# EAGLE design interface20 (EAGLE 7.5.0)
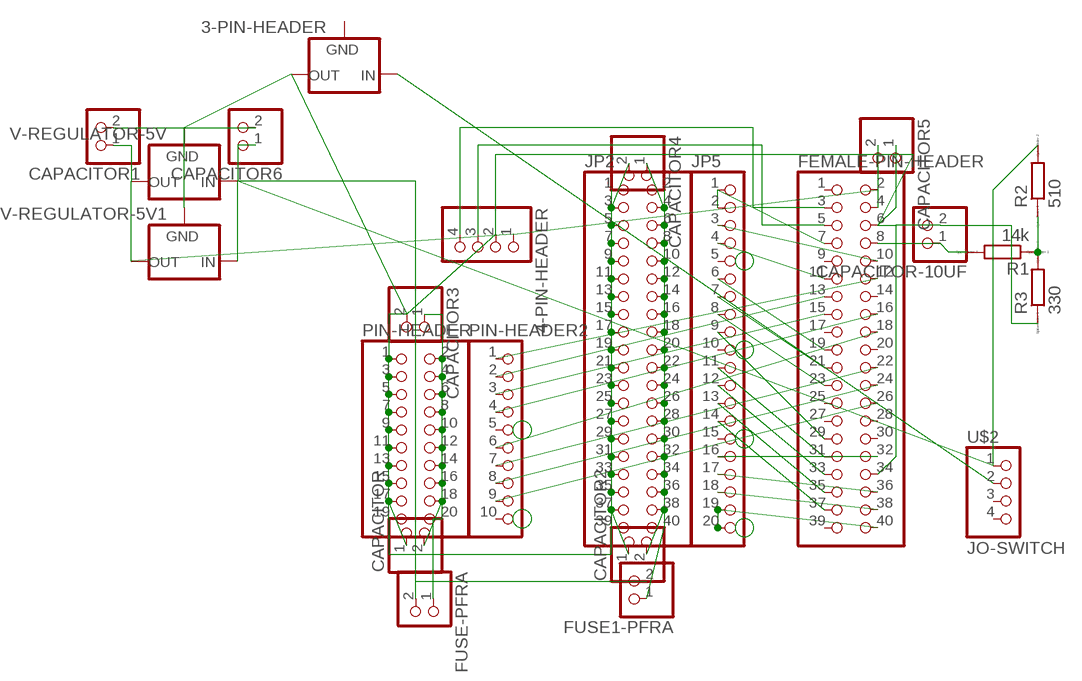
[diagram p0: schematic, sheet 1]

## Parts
3-PIN-HEADER  78MXXS  [78MXXS]
4-PIN-HEADER  PINHD-1X4  [1X04]
CAPACITOR  PINHD-1X2  [1X02]
CAPACITOR1  PINHD-1X2  [1X02]
CAPACITOR2  PINHD-1X2  [1X02]
CAPACITOR3  PINHD-1X2  [1X02]
CAPACITOR4  PINHD-1X2  [1X02]
CAPACITOR5  PINHD-1X2  [1X02]
CAPACITOR6  PINHD-1X2  [1X02]
CAPACITOR-10UF  PINHD-1X2  [1X02]
FEMALE-PIN-HEADER  PINHD-2X20  [2X20]
FUSE1-PFRA  PINHD-1X2  [1X02]
FUSE-PFRA  PINHD-1X2  [1X02]
JP2  PINHD-2X20  [2X20]
JP5  PINHD-1X20  [1X20]
PIN-HEADER  PINHD-2X10  [2X10]
PIN-HEADER2  PINHD-1X10  [1X10]
R1  14k  R0204/7  [0204/7]
R2  510  R0204/7  [0204/7]
R3  330  R0204/7  [0204/7]
U$2  JO-SWITCH  [JO-SWICH]
V-REGULATOR-5V  78MXXS  [78MXXS]
V-REGULATOR-5V1  78MXXS  [78MXXS]

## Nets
N$1 [dicker]: 3-PIN-HEADER.IN U$2.2
N$2: CAPACITOR-10UF.1 FEMALE-PIN-HEADER.8 R1.2
N$4: R1.1 R2.1 R3.2
N$7: 4-PIN-HEADER.4 FEMALE-PIN-HEADER.3
N$8: 4-PIN-HEADER.3 FEMALE-PIN-HEADER.5
N$9: FEMALE-PIN-HEADER.7 JP5.1 JP5.2
N$10: FEMALE-PIN-HEADER.10 JP5.3
N$11: FEMALE-PIN-HEADER.13 PIN-HEADER2.2
N$12: FEMALE-PIN-HEADER.11 JP5.4
N$13: FEMALE-PIN-HEADER.19 JP5.6
N$14: FEMALE-PIN-HEADER.21 JP5.7
N$15: FEMALE-PIN-HEADER.23 JP5.8
N$16: FEMALE-PIN-HEADER.29 JP5.9
N$17: FEMALE-PIN-HEADER.31 JP5.11
N$18: FEMALE-PIN-HEADER.33 JP5.12
N$19: FEMALE-PIN-HEADER.35 JP5.13
N$20: FEMALE-PIN-HEADER.37 JP5.14
N$21: FEMALE-PIN-HEADER.40 JP5.19 JP5.20
N$22: FEMALE-PIN-HEADER.38 JP5.18
N$23: FEMALE-PIN-HEADER.36 JP5.17
N$24: FEMALE-PIN-HEADER.32 JP5.16
N$25: FEMALE-PIN-HEADER.26 PIN-HEADER2.9
N$26: FEMALE-PIN-HEADER.24 PIN-HEADER2.8
N$27: FEMALE-PIN-HEADER.22 PIN-HEADER2.7
N$28: FEMALE-PIN-HEADER.18 PIN-HEADER2.6
N$29: FEMALE-PIN-HEADER.16 PIN-HEADER2.4
N$30: FEMALE-PIN-HEADER.12 PIN-HEADER2.1
N$31: FEMALE-PIN-HEADER.15 PIN-HEADER2.3
N$32 [mittel]: 4-PIN-HEADER.1 CAPACITOR1.1 CAPACITOR5.2 FEMALE-PIN-HEADER.2 FEMALE-PIN-HEADER.4 V-REGULATOR-5V1.OUT V-REGULATOR-5V.OUT
N$33 [dicker]: 3-PIN-HEADER.OUT 4-PIN-HEADER.2 CAPACITOR1.2 CAPACITOR2.1 CAPACITOR3.2 CAPACITOR4.2 CAPACITOR5.1 CAPACITOR6.2 CAPACITOR-10UF.2 CAPACITOR.1 FEMALE-PIN-HEADER.6 FEMALE-PIN-HEADER.34 JP2.1 JP2.3 JP2.5 JP2.7 JP2.9 JP2.11 JP2.13 JP2.15 JP2.17 JP2.19 JP2.21 JP2.23 JP2.25 JP2.27 JP2.29 JP2.31 JP2.33 JP2.35 JP2.37 JP2.39 PIN-HEADER.1 PIN-HEADER.3 PIN-HEADER.5 PIN-HEADER.7 PIN-HEADER.9 PIN-HEADER.11 PIN-HEADER.13 PIN-HEADER.15 PIN-HEADER.17 PIN-HEADER.19 R3.1 V-REGULATOR-5V1.GND V-REGULATOR-5V.GND
N$35 [dicker]: CAPACITOR2.2 CAPACITOR4.1 FUSE1-PFRA.1 JP2.2 JP2.4 JP2.6 JP2.8 JP2.10 JP2.12 JP2.14 JP2.16 JP2.18 JP2.20 JP2.22 JP2.24 JP2.26 JP2.28 JP2.30 JP2.32 JP2.34 JP2.36 JP2.38 JP2.40
N$36 [dicker]: CAPACITOR6.1 FUSE1-PFRA.2 FUSE-PFRA.2 R2.2 U$2.1 V-REGULATOR-5V1.IN V-REGULATOR-5V.IN
N$37 [dicker]: CAPACITOR3.1 CAPACITOR.2 FUSE-PFRA.1 PIN-HEADER.2 PIN-HEADER.4 PIN-HEADER.6 PIN-HEADER.8 PIN-HEADER.10 PIN-HEADER.12 PIN-HEADER.14 PIN-HEADER.16 PIN-HEADER.18 PIN-HEADER.20
Unconnected: 3-PIN-HEADER.GND FEMALE-PIN-HEADER.1 FEMALE-PIN-HEADER.9 FEMALE-PIN-HEADER.14 FEMALE-PIN-HEADER.17 FEMALE-PIN-HEADER.20 FEMALE-PIN-HEADER.25 FEMALE-PIN-HEADER.27 FEMALE-PIN-HEADER.28 FEMALE-PIN-HEADER.30 FEMALE-PIN-HEADER.39 JP5.5 JP5.10 JP5.15 PIN-HEADER2.5 PIN-HEADER2.10 U$2.3 U$2.4

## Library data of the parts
3-PIN-HEADER V-REGULATOR-5V V-REGULATOR-5V1 = v-reg:78MXXS: VOLTAGE REGULATOR
4-PIN-HEADER = pinhead:PINHD-1X4: PIN HEADER
CAPACITOR CAPACITOR1-CAPACITOR6 CAPACITOR-10UF FUSE1-PFRA FUSE-PFRA = pinhead:PINHD-1X2: PIN HEADER
FEMALE-PIN-HEADER JP2 = pinhead:PINHD-2X20: PIN HEADER
JP5 = pinhead:PINHD-1X20: PIN HEADER
PIN-HEADER = pinhead:PINHD-2X10: PIN HEADER
PIN-HEADER2 = pinhead:PINHD-1X10: PIN HEADER
R1-R3 = eagle-ltspice:R: RESISTOR, European symbol; SPICEMODEL: NONE; SPICEPREFIX: R
U$2 = pinhead:JO-SWITCH

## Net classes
1 dicker: width 1.27 mm, drill 1.016 mm, clearance 0.127 mm
2 mittel: width 0.508 mm, drill 0.508 mm

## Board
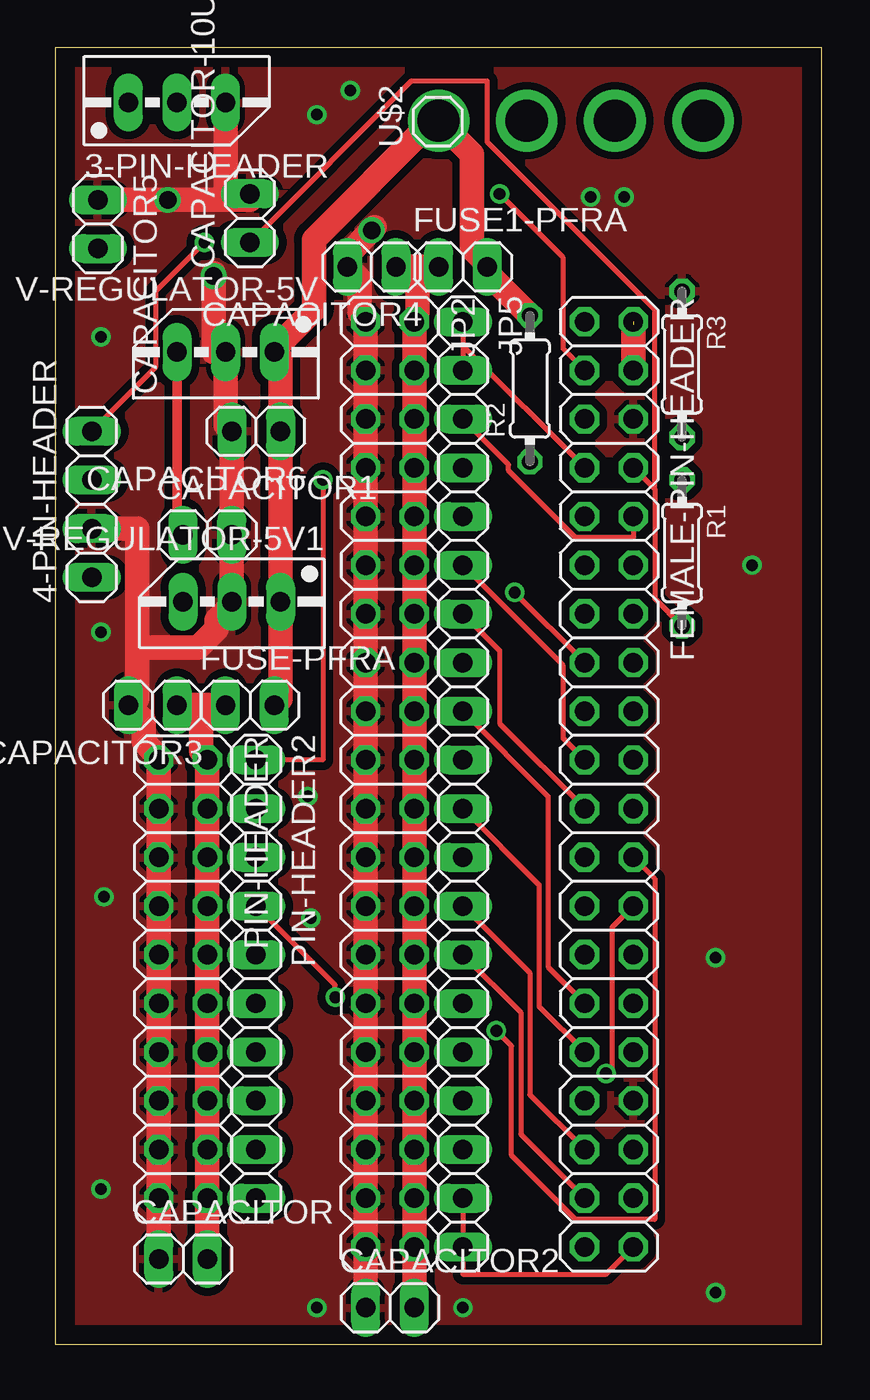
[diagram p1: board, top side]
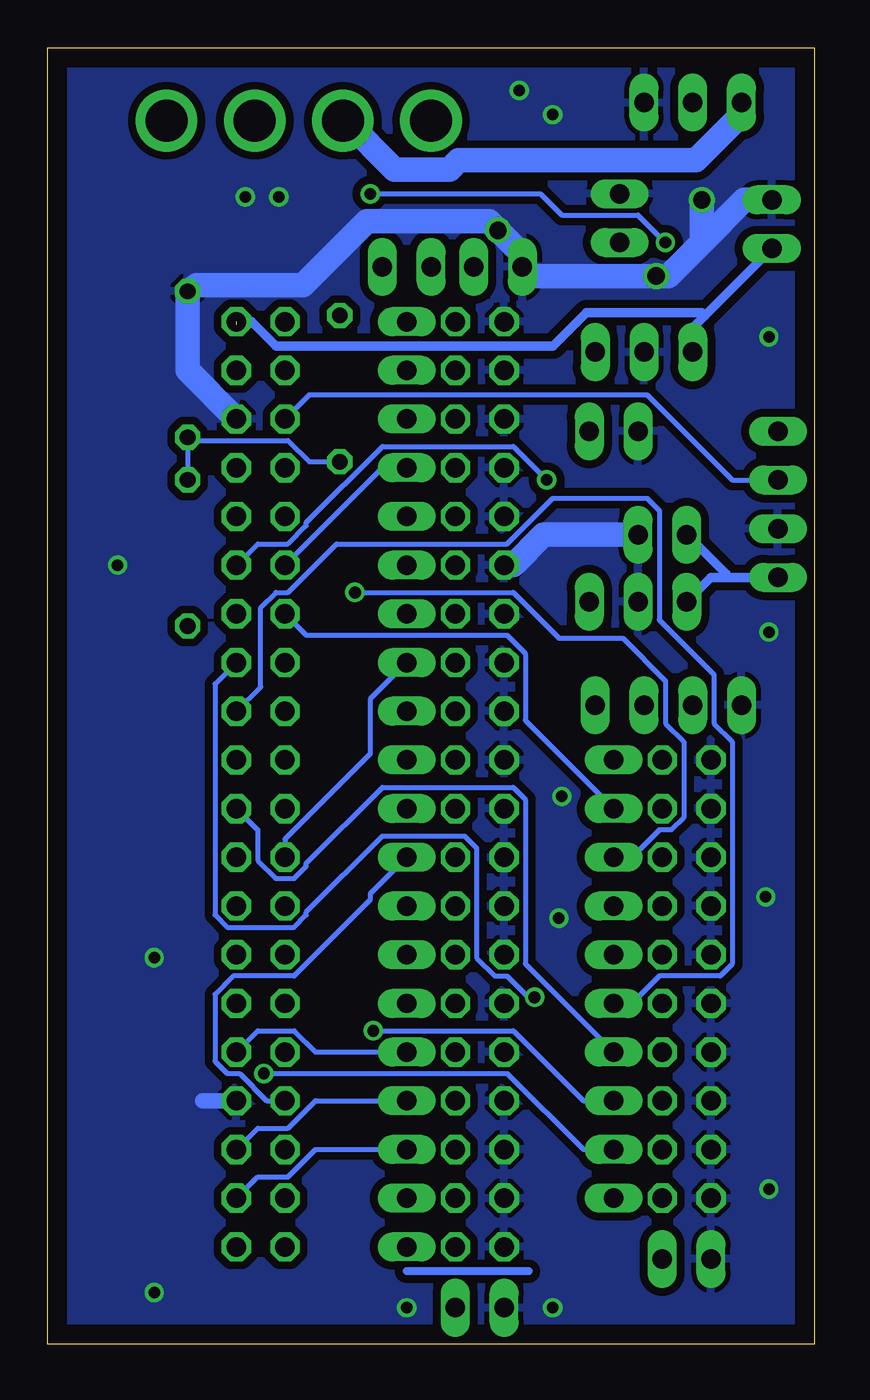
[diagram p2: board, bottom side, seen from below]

Size 39.99 x 67.62 mm. Coordinates in mm from the lower left corner, seen from the top.
Outline: 0,0 39.99,0 39.99,67.62 0,67.62 0,0
Copper layers (1*16): Top 0.035mm / dielectric 1.5mm / Bottom 0.035mm
Design rules "default *": minimum track width 10mil, minimum drill 24mil, track to track 8mil, track to pad 8mil, pad to pad 8mil, via to via 8mil, smd to smd 8mil, copper to edge 40mil, drill to drill 8mil, minimum pad ring 10mil, minimum via ring 8mil, stop-mask expansion 4mil, vias tented up to drill 0mil, thermal gap 10mil

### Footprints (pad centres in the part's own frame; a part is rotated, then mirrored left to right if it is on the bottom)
78MXXS = drill 1.016 long: GND 0,-2.54; IN -2.54,-2.54; OUT 2.54,-2.54
1X04 = drill 1.016 pad 1.194 long: 1 -3.81,0; 2 -1.27,0; 3 1.27,0; 4 3.81,0
1X02 = drill 1.016 long: 1 -1.27,0; 2 1.27,0
2X20 = drill 1.016 octagon: 1 -24.13,-1.27; 2 -24.13,1.27; 3 -21.59,-1.27; 4 -21.59,1.27; 5 -19.05,-1.27; 6 -19.05,1.27; 7 -16.51,-1.27; 8 -16.51,1.27; 9 -13.97,-1.27; 10 -13.97,1.27; 11 -11.43,-1.27; 12 -11.43,1.27; 13 -8.89,-1.27; 14 -8.89,1.27; 15 -6.35,-1.27; 16 -6.35,1.27; 17 -3.81,-1.27; 18 -3.81,1.27; 19 -1.27,-1.27; 20 -1.27,1.27; 21 1.27,-1.27; 22 1.27,1.27; 23 3.81,-1.27; 24 3.81,1.27; 25 6.35,-1.27; 26 6.35,1.27; 27 8.89,-1.27; 28 8.89,1.27; 29 11.43,-1.27; 30 11.43,1.27; 31 13.97,-1.27; 32 13.97,1.27; 33 16.51,-1.27; 34 16.51,1.27; 35 19.05,-1.27; 36 19.05,1.27; 37 21.59,-1.27; 38 21.59,1.27; 39 24.13,-1.27; 40 24.13,1.27
1X20 = drill 1.016 long: 1 -24.13,0; 2 -21.59,0; 3 -19.05,0; 4 -16.51,0; 5 -13.97,0; 6 -11.43,0; 7 -8.89,0; 8 -6.35,0; 9 -3.81,0; 10 -1.27,0; 11 1.27,0; 12 3.81,0; 13 6.35,0; 14 8.89,0; 15 11.43,0; 16 13.97,0; 17 16.51,0; 18 19.05,0; 19 21.59,0; 20 24.13,0
2X10 = drill 1.016 octagon: 1 -11.43,-1.27; 2 -11.43,1.27; 3 -8.89,-1.27; 4 -8.89,1.27; 5 -6.35,-1.27; 6 -6.35,1.27; 7 -3.81,-1.27; 8 -3.81,1.27; 9 -1.27,-1.27; 10 -1.27,1.27; 11 1.27,-1.27; 12 1.27,1.27; 13 3.81,-1.27; 14 3.81,1.27; 15 6.35,-1.27; 16 6.35,1.27; 17 8.89,-1.27; 18 8.89,1.27; 19 11.43,-1.27; 20 11.43,1.27
1X10 = drill 1.016 long: 1 -11.43,0; 2 -8.89,0; 3 -6.35,0; 4 -3.81,0; 5 -1.27,0; 6 1.27,0; 7 3.81,0; 8 6.35,0; 9 8.89,0; 10 11.43,0
0204/7 = drill 0.813 octagon: 1 -3.81,0; 2 3.81,0
JO-SWICH = drill 2.2: 1 0,0; 2 0,-4.6; 3 0,-9.2; 4 0,-13.8

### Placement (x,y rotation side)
3-PIN-HEADER  6.35,67.31 0 top
4-PIN-HEADER  1.91,43.82 90 top
CAPACITOR  6.67,4.45 0 top
CAPACITOR1  7.94,42.23 0 top
CAPACITOR2  17.46,1.91 0 top
CAPACITOR3  5.08,33.34 180 top
CAPACITOR4  16.51,56.2 180 top
CAPACITOR5  2.22,58.42 270 top
CAPACITOR6  10.48,47.62 180 top
CAPACITOR-10UF  10.16,58.74 90 top
FEMALE-PIN-HEADER  28.89,29.21 270 top
FUSE1-PFRA  21.27,56.2 0 top
FUSE-PFRA  10.16,33.34 0 top
JP2  17.46,29.21 270 top
JP5  21.27,29.21 270 top
PIN-HEADER  6.67,19.05 270 top
PIN-HEADER2  10.48,19.05 270 top
R1  32.7,41.28 270 top
R2  24.77,49.85 90 top
R3  32.7,51.12 270 top
U$2  20,63.82 90 top
V-REGULATOR-5V  8.89,49.21 180 top
V-REGULATOR-5V1  9.21,36.2 180 top

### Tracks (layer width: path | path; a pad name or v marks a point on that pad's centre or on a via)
N$1
  Bottom 1.27: 3-PIN-HEADER.IN 3.81,64.14 6.19,61.75 18.57,61.75 19.05,61.28 21.91,61.28 24.45,63.82 U$2.2
N$2
  Top 0.254: R1.2 31.27,38.89 31.27,44.61 31.19,44.69 | FEMALE-PIN-HEADER.8 31.19,44.69 | CAPACITOR-10UF.1 18.57,65.88 22.54,65.88 22.54,62.71 31.27,53.98 31.27,44.77 31.19,44.69
N$3
  Bottom 0.406: 14.92,3.81 21.27,3.81
N$4
  Bottom 0.254: R2.1 26.35,46.04 27.46,47.15 32.54,47.15 R3.2 R1.1
N$7  (via drill 0.61)
  Top 0.254: 4-PIN-HEADER.4 5.24,50.96 5.24,54.93 v7.78,57.47 | v23.18,60.01 26.51,56.67 26.51,51.91 FEMALE-PIN-HEADER.3
  Bottom 0.254: v7.78,57.47 9.21,58.9 13.18,58.9 14.29,60.01 v23.18,60.01
N$8
  Bottom 0.254: 4-PIN-HEADER.3 4.29,45.09 8.73,49.53 26.35,49.53 FEMALE-PIN-HEADER.5
N$9
  Top 0.254: JP5.1 21.27,52.07 | 21.27,52.07 JP5.2 | 21.27,52.07 FEMALE-PIN-HEADER.7
N$10
  Top 0.254: JP5.3 23.65,45.88 23.65,45.56 27.15,42.07 30.16,42.07 FEMALE-PIN-HEADER.10
N$11
  Bottom 0.254: PIN-HEADER2.2 15.08,32.54 15.08,36.04 16.03,36.99 26.51,36.99 FEMALE-PIN-HEADER.13
N$12
  Bottom 0.254: JP5.4 22.54,45.72 FEMALE-PIN-HEADER.11
N$13
  Top 0.254: JP5.6 26.51,35.4 26.51,31.59 FEMALE-PIN-HEADER.19
N$14
  Top 0.254: FEMALE-PIN-HEADER.21 23.18,32.38 23.18,36.2 JP5.7
N$15
  Bottom 0.254: FEMALE-PIN-HEADER.23 27.62,26.35 23.18,30.8 23.18,33.66 JP5.8
N$16
  Top 0.254: FEMALE-PIN-HEADER.29 25.72,19.68 25.72,28.57 JP5.9
N$17
  Top 0.254: FEMALE-PIN-HEADER.31 25.24,17.62 25.24,23.97 JP5.11
N$18
  Bottom 0.254: FEMALE-PIN-HEADER.33 28.58,12.7 30,14.13 30.64,14.13 31.27,14.76 31.27,18.26 30.32,19.21 27.15,19.21 23.18,23.18 23.18,23.5 JP5.12
N$19
  Top 0.254: FEMALE-PIN-HEADER.35 24.76,13.02 24.76,19.37 JP5.13
N$20
  Top 0.254: FEMALE-PIN-HEADER.37 24.29,10.95 24.29,17.3 JP5.14
N$21
  Top 0.254: JP5.19 JP5.20 21.27,3.65 28.73,3.65 FEMALE-PIN-HEADER.40
N$22
  Bottom 0.254: JP5.18 26.04,10.16 27.46,8.73 29.05,8.73 FEMALE-PIN-HEADER.38
N$23
  Bottom 0.254: JP5.17 26.04,12.7 27.46,11.27 29.05,11.27 FEMALE-PIN-HEADER.36
N$24
  Bottom 0.254: JP5.16 26.04,15.24 27.15,16.35 29.05,16.35 FEMALE-PIN-HEADER.32
N$25  (via drill 0.61)
  Top 0.254: v28.73,14.13 29.05,14.45 29.05,21.75 FEMALE-PIN-HEADER.26
  Bottom 0.254: PIN-HEADER2.9 12.06,10.16 16.03,14.13 v28.73,14.13
N$26  (via drill 0.61)
  Top 0.254: v23.02,16.35 23.81,15.56 23.81,9.84 27.15,6.51 31.27,6.51 31.27,24.29 FEMALE-PIN-HEADER.24
  Bottom 0.254: PIN-HEADER2.8 12.06,12.7 15.72,16.35 v23.02,16.35
N$27
  Bottom 0.254: PIN-HEADER2.7 15.08,19.84 15.08,28.42 15.72,29.05 22.54,29.05 26.51,25.08 26.51,24.92 27.15,24.29 28.1,24.29 29.05,25.24 29.05,26.83 FEMALE-PIN-HEADER.22
N$28
  Bottom 0.254: PIN-HEADER2.6 9.53,17.78 8.1,19.21 4.92,19.21 4.29,19.84 4.29,31.43 5.24,32.38 5.24,34.93 8.1,37.78 8.1,43.5 8.73,44.13 13.65,44.13 16.03,41.75 24.92,41.75 27.46,39.21 28.1,39.21 28.89,38.42 28.89,34.29 FEMALE-PIN-HEADER.18
N$29  (via drill 0.61)
  Top 0.254: PIN-HEADER2.4 14.61,18.73 v14.61,18.1
  Bottom 0.254: v14.61,18.1 14.92,18.1 16.03,19.21 16.67,19.21 17.62,20.16 17.62,25.88 18.26,26.51 22.54,26.51 26.51,22.54 26.51,22.38 27.15,21.75 30.64,21.75 31.27,22.38 31.27,34.45 FEMALE-PIN-HEADER.16
N$30  (via drill 0.61)
  Top 0.254: PIN-HEADER2.1 13.97,30.48 v13.97,45.09
  Bottom 0.254: v13.97,45.09 15.72,46.83 22.54,46.83 26.51,42.86 26.51,42.7 27.46,41.75 29.05,41.75 FEMALE-PIN-HEADER.12
N$31  (via drill 0.61)
  Top 0.254: FEMALE-PIN-HEADER.15 v23.97,39.21
  Bottom 0.254: PIN-HEADER2.3 9.53,25.4 8.1,26.83 7.46,26.83 6.83,27.46 6.83,31.43 7.78,32.38 7.78,34.61 10,36.83 13.33,36.83 15.72,39.21 v23.97,39.21
N$32  (1 unrouted)
  Top 0.508: CAPACITOR1.1 6.35,42.55 V-REGULATOR-5V.OUT
  Top 1.27: FEMALE-PIN-HEADER.4 30.16,53.18
  Bottom 0.508: 4.6,40.01 5.4,40.01 V-REGULATOR-5V1.OUT | 4.6,40.01 4-PIN-HEADER.1 | CAPACITOR1.1 4.6,40.16 4.6,40.01 | V-REGULATOR-5V.OUT 6.35,53.02 5.71,53.66 | CAPACITOR5.2 5.71,53.66 | FEMALE-PIN-HEADER.2 29.37,53.34 28.1,52.07 13.65,52.07 11.91,53.82 5.87,53.82 5.71,53.66
N$33  (via drill 0.6, 0.9)
  Top 1.27: CAPACITOR.1 PIN-HEADER.19 PIN-HEADER.17 PIN-HEADER.15 PIN-HEADER.13 PIN-HEADER.11 PIN-HEADER.9 PIN-HEADER.7 PIN-HEADER.5 PIN-HEADER.3 PIN-HEADER.1 5.08,30.96 4.6,31.43 4.6,32.54 CAPACITOR3.2 4.29,33.66 4.29,36.35 | 4-PIN-HEADER.2 4.29,42.55 4.29,36.35 | 4.29,36.35 7.46,36.35 8.41,37.31 8.41,37.78 8.89,38.26 V-REGULATOR-5V1.GND CAPACITOR1.2 CAPACITOR6.2 8.89,47.94 V-REGULATOR-5V.GND 8.26,51.75 v8.26,55.72 8.26,55.88 | CAPACITOR5.1 v5.87,59.69 10.16,59.69 CAPACITOR-10UF.2 8.89,60.17 3-PIN-HEADER.OUT | CAPACITOR2.1 JP2.39 JP2.37 JP2.35 JP2.33 JP2.31 JP2.29 JP2.27 JP2.25 JP2.23 JP2.21 JP2.19 JP2.17 JP2.15 JP2.13 JP2.11 JP2.9 JP2.7 JP2.5 JP2.3 JP2.1 15.87,53.82 15.87,55.56 CAPACITOR4.2 15.24,56.83 v16.51,58.1 16.67,58.26
  Bottom 0.813: FEMALE-PIN-HEADER.34 31.91,12.7
  Bottom 1.27: FEMALE-PIN-HEADER.6 32.7,50.8 R3.1 32.23,55.25 26.67,55.25 23.34,58.58 16.99,58.58 v16.51,58.1 15.24,56.83 CAPACITOR4.2 14.92,55.72 v8.26,55.72 7.62,55.72 5.87,57.47 | CAPACITOR5.1 3.65,59.69 5.87,57.47 | CAPACITOR1.2 14.13,42.23 15.72,40.64 JP2.11 | v5.87,59.69 5.87,57.47
  other vias: 21.27,1.91 34.45,2.7 34.45,20.16 13.65,1.91 2.38,8.1 2.54,23.34 2.38,37.15 36.35,40.64 13.34,22.22 13.18,28.57 29.69,59.85 27.94,59.85 15.4,65.41 13.65,64.14 2.38,52.55
  pour Bottom (isolate 0.406): 0,67.79 0,0 40.32,0 40.32,67.15 39.85,67.63 0.32,67.63 0,67.94
  pour Top (isolate 0.406): 0,67.79 0,0.16 0.16,0 40.01,0 40.01,67.94 0,67.94
N$35
  Top 1.27: FUSE1-PFRA.1 18.89,56.2 | 18.89,56.2 CAPACITOR4.1 | CAPACITOR2.2 JP2.40 JP2.38 JP2.36 JP2.34 JP2.32 JP2.30 JP2.28 JP2.26 JP2.24 JP2.22 JP2.20 JP2.18 JP2.16 JP2.14 JP2.12 JP2.10 JP2.8 JP2.6 JP2.4 JP2.2 18.89,53.82 18.89,56.2
N$36
  Top 1.27: FUSE-PFRA.2 11.75,33.66 V-REGULATOR-5V1.IN CAPACITOR6.1 11.75,51.44 V-REGULATOR-5V.IN 11.75,52.23 13.49,53.98 13.49,57.63 19.53,63.66 U$2.1 21.75,62.07 21.75,57.15 22.23,56.67 FUSE1-PFRA.2 22.54,55.88 R2.2
N$37
  Top 1.27: FUSE-PFRA.1 7.62,33.34 | 7.62,33.34 CAPACITOR3.1 | CAPACITOR.2 PIN-HEADER.20 PIN-HEADER.18 PIN-HEADER.16 PIN-HEADER.14 PIN-HEADER.12 PIN-HEADER.10 PIN-HEADER.8 PIN-HEADER.6 PIN-HEADER.4 PIN-HEADER.2 7.62,30.96 7.62,33.34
